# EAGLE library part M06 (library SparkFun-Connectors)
Header 6 Standard 6-pin 0.1" header. Use with straight break away headers (SKU : PRT-00116), right angle break away headers (PRT-00553), swiss pins (PRT-00743), machine pins (PRT-00117), and female headers (PRT-00115). Molex polarized connector foot print use with SKU : PRT-08094 with associated crimp pins and housings. NOTES ON THE VARIANTS LOCK and LOCK_LONGPADS... This footprint was designed to help hold the alignment of a through-hole component (i.e. 6-pin header) while soldering it into place. You may notice that each hole has been shifted either up or down by 0.005 of an inch from it's more standard position (which is a perfectly straight line). This slight alteration caused the pins (the squares in the middle) to touch the edges of the holes. Because they are alternating, it causes a "brace" to hold the component in place. 0.005 has proven to be the perfect amount of "off-center" position when using our standard breakaway headers. Although looks a little odd when you look at the bare footprint, once you have a header in there, the alteration is very hard to notice. Also,if you push a header all the way into place, it is covered up entirely on the bottom side. This idea of altering the position of holes to aid alignment will be further integrated into the Sparkfun Library for other footprints. It can help hold any component with 3 or more connection pins.
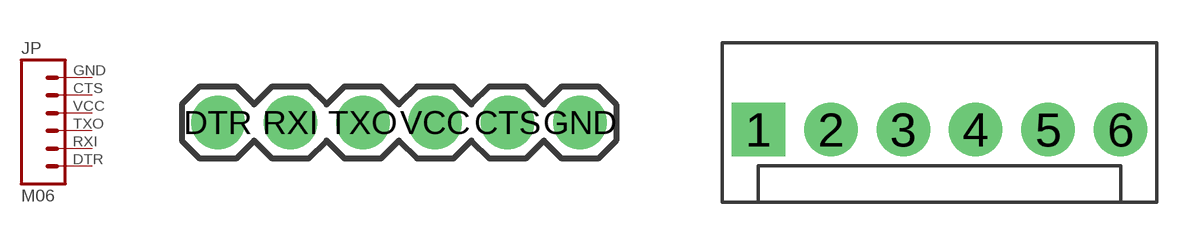
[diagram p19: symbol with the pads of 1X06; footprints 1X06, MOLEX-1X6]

Designator prefix JP

## M06SIP  [1X06]
CTS  5  pas
DTR  1  pas
GND  6  pas
RXI  2  pas
TXO  3  pas
VCC  4  pas

## M06POLAR  [MOLEX-1X6]
1  1  pas
2  2  pas
3  3  pas
4  4  pas
5  5  pas
6  6  pas

## M06RA  [MOLEX-1X6-RA]
Pads as for MOLEX-1X6

## M06SMD  [1X06-SMD]
Pads as for MOLEX-1X6

## M06LOCK  [1X06_LOCK]
Pads as for MOLEX-1X6

## M06LOCK_LONGPADS  [1X06_LOCK_LONGPADS]
Pads as for MOLEX-1X6

## M06POLAR_LOCK  [MOLEX-1X6_LOCK]
Pads as for MOLEX-1X6

## M06RA_LOCK  [MOLEX-1X6-RA_LOCK]
Pads as for MOLEX-1X6

## M06SIP_LOCK  [1X06-SIP_LOCK]
Pads as for MOLEX-1X6

## M06FEMALE_LOCK  [1X06_FEMALE_LOCK.010]
Pads as for MOLEX-1X6

## M06LONGPADS  [1X06_LONGPADS]
Pads as for MOLEX-1X6

## M061X06-SMD_EDGE_FEMALE  [1X06-SMD_EDGE]
Pads as for MOLEX-1X6

## M063.5MM-6  [SCREWTERMINAL-3.5MM-6]
Pads as for MOLEX-1X6

## M06SMDF  [1X06-SMD-FEMALE]
Pads as for MOLEX-1X6

## M06SMD-FEMALE-V2  [1X06-SMD-FEMALE-V2]
Pads as for MOLEX-1X6

## M06POGOPIN_HOLES_ONLY  [1X06_HOLES_ONLY]
Pads as for MOLEX-1X6

## M06SMD-STRAIGHT  [1X06_SMD_STRAIGHT]
Pads as for MOLEX-1X6

## M06SMD-STRAIGHT-ALT  [1X06_SMD_STRAIGHT_ALT]
Pads as for MOLEX-1X6

## M06SMD-STRAIGHT-COMBO  [1X06_SMD_STRAIGHT_COMBO]
Pads as for MOLEX-1X6

## M06VERNIER-ANALOG  [BTA]
Pads as for MOLEX-1X6

## M06VERNIER-DIGITAL  [BTD]
Pads as for MOLEX-1X6

## M06SMD_MALE (PROD_ID: CONN-11293)  [1X06_SMD_MALE]
Pads as for MOLEX-1X6

## M06SMD-1MM  [1X06-1MM]
Pads as for MOLEX-1X6

## M06NO_SILK  [1X06_NO_SILK]
Pads as for MOLEX-1X6

## Footprint 1X06 (pad centres in mm)
drill 1.016 pad 1.88: CTS 10.16,0; DTR 0,0; GND 12.7,0; RXI 2.54,0; TXO 5.08,0; VCC 7.62,0

## Footprint MOLEX-1X6 (pad centres in mm)
drill 1.016 pad 1.88 square: 1 0,0
drill 1.016 pad 1.88: 2 2.54,0; 3 5.08,0; 4 7.62,0; 5 10.16,0; 6 12.7,0

## Footprint MOLEX-1X6-RA (pad centres in mm)
drill 1.016 pad 1.88 square: 1 0,0
drill 1.016 pad 1.88: 2 2.54,0; 3 5.08,0; 4 7.62,0; 5 10.16,0; 6 12.7,0

## Footprint 1X06-SMD (pad centres in mm)
smd 1 x 3: 1 -6.35,5; 2 -3.81,5; 3 -1.27,5; 4 1.27,5; 5 3.81,5; 6 6.35,5
hole 1.4 at -5.08,0
hole 1.4 at 5.08,0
